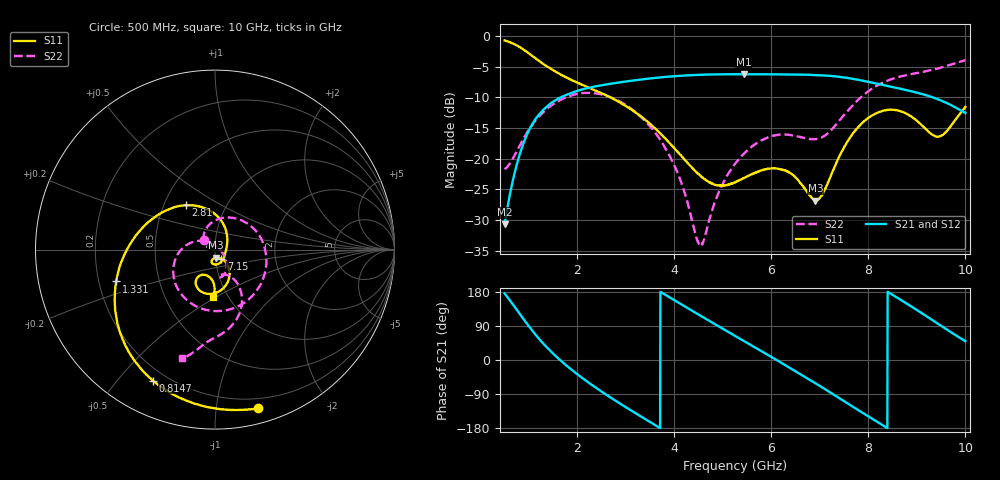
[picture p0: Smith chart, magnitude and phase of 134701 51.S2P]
!  2-Port S-parameters saved by WinCal
! VAR MeasName=S-Parameters (CALIBRATED_DATA) read from VNA (N5242A)
! VAR MeasDate=2013-7-3 16:39:38
! VAR NAME=134701 51
! VAR FILENAME=134701 51.S2P
! VAR DATE=2013-7-3 16:39:38
! VAR PHYS_PORTS=1,2
# Hz S MA R 50
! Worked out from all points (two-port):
!   1601 points, 500 MHz to 10 GHz, reference 50 ohm
!   highest |S21| = -6.24 dB at 5.434 GHz (marker M1); lowest = -30.7 dB at 500 MHz (marker M2)
!   |S21| within 3 dB of the highest: 1.894 GHz to 8.997 GHz (7.102 GHz wide, 130 % of centre)
!   lowest |S11| = -26.8 dB at 6.907 GHz (marker M3), VSWR 1.10, Z = 50.2 - j4.56 ohm
!   |S11| at or under -10 dB: 2.676 GHz to end of sweep
!   |S22| runs from -34.3 to -4.0 dB; largest |S21 - S12| = 0.0024
!   S11 on the Smith chart (normalised r, x): 500 MHz: 0.12, -1.30; 814.7 MHz: 0.15, -0.62; 1.331 GHz: 0.27, -0.15; 2.81 GHz: 0.64, +0.35; 7.15 GHz: 1.07, -0.11; 10 GHz: 0.85, -0.48
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5e8  0.9169 -74.7  0.02915 175.5  0.02927 175.3  0.08207 140.8
8.146875e8  0.8078 -115.3  0.1095 121.3  0.1095 121.2  0.1282 112.1
1.034375e9  0.7039 -138.6  0.1801 83.4  0.18 83.3  0.1803 77.0
1.33125e9  0.5783 -162.2  0.2571 38.7  0.2569 38.6  0.2458 27.6
1.675625e9  0.4795 177.5  0.3179 -3.8  0.3178 -3.9  0.3035 -21.6
2.085312e9  0.4021 157.6  0.3648 -46.0  0.3642 -46.1  0.3413 -69.0
2.809688e9  0.2968 123.6  0.4144 -109.3  0.4134 -109.4  0.3008 -133.7
3.670625e9  0.1666 78.3  0.4574 -177.0  0.4566 -176.9  0.1496 167.4
4.080312e9  0.112 54.5  0.4713 151.7  0.471 151.7  0.0742 140.3
4.5375e9  0.07243 22.7  0.4817 117.0  0.4816 117.1  0.01938 47.6
4.929375e9  0.06051 -10.1  0.4861 87.6  0.4862 87.7  0.05482 -29.9
5.25e9  0.06407 -36.9  0.4869 63.7  0.4873 63.7  0.09086 -46.3
5.434062e9  0.06946 -50.6  0.4874 50.0  0.4869 50.0  0.1098 -53.4
6.134688e9  0.08293 -92.0  0.4854 -2.1  0.4858 -2.1  0.1559 -75.9
6.835312e9  0.04791 -94.7  0.4813 -55.7  0.4814 -55.6  0.1438 -77.2
6.906562e9  0.04552 -85.4  0.4797 -61.2  0.4799 -61.2  0.1442 -74.3
7.15e9  0.06145 -55.9  0.4738 -80.6  0.4739 -80.6  0.1592 -63.7
7.749688e9  0.1735 -62.7  0.441 -128.9  0.4421 -129.0  0.2909 -59.4
8.420625e9  0.2496 -98.6  0.3884 178.0  0.3885 177.9  0.4358 -78.1
8.966875e9  0.2083 -121.0  0.3469 134.6  0.3469 134.3  0.4951 -91.1
9.43e9  0.1511 -109.0  0.3049 96.0  0.3049 95.8  0.5423 -97.9
1e10  0.2636 -92.5  0.2354 49.6  0.2351 49.4  0.633 -106.8
